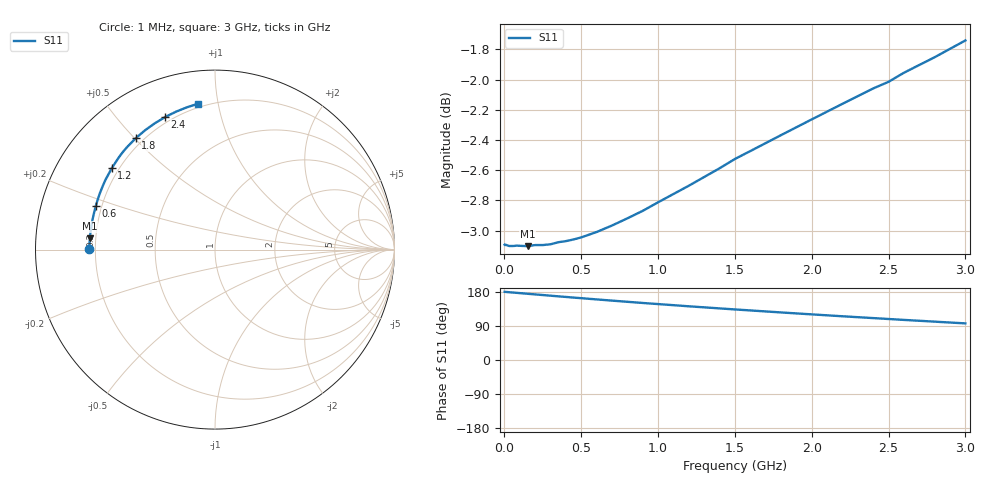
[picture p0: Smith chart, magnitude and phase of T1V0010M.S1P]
! SIEMENS Small Signal Semiconductors
! BAT68-04
! Si Schottky Diode (2 diodes in series, pin 3 open) in SOT23
! IF = 10 mA
! S-Parameters:  August  1994
# GHz  S  MA  R  50
!  f  S11
! GHz  MAG  ANG
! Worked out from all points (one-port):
!   33 points, 1 MHz to 3 GHz, reference 50 ohm
!   lowest |S11| = -3.1 dB at 150 MHz (marker M1), VSWR 5.66, Z = 8.86 + j2.2 ohm
!   |S11| at or under -10 dB: nowhere
!   S11 on the Smith chart (normalised r, x): 1 MHz: 0.18, +0.00; 600 MHz: 0.18, +0.17; 1.2 GHz: 0.17, +0.34; 1.8 GHz: 0.17, +0.50; 2.4 GHz: 0.17, +0.68; 3 GHz: 0.18, +0.88
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0.001  0.7004 179.9
0.003  0.7002 179.8
0.01  0.7003 179.6
0.03  0.6997 178.9
0.08  0.6999 177.2
0.15  0.6996 174.8
0.2  0.7002 173.1
0.25  0.7002 171.4
0.35  0.7017 168.0
0.4  0.7023 166.4
0.45  0.7032 164.7
0.6  0.7072 159.9
0.7  0.7107 156.7
0.8  0.7146 153.6
0.9  0.7187 150.5
1  0.7234 147.6
1.2  0.7326 141.7
1.4  0.7424 136.2
1.5  0.7477 133.4
1.6  0.7522 130.8
1.8  0.7614 125.5
2  0.7706 120.4
2.2  0.7798 115.4
2.4  0.789 110.6
2.5  0.793 108.2
2.6  0.7985 105.8
2.8  0.808 101.2
3  0.8184 96.6
